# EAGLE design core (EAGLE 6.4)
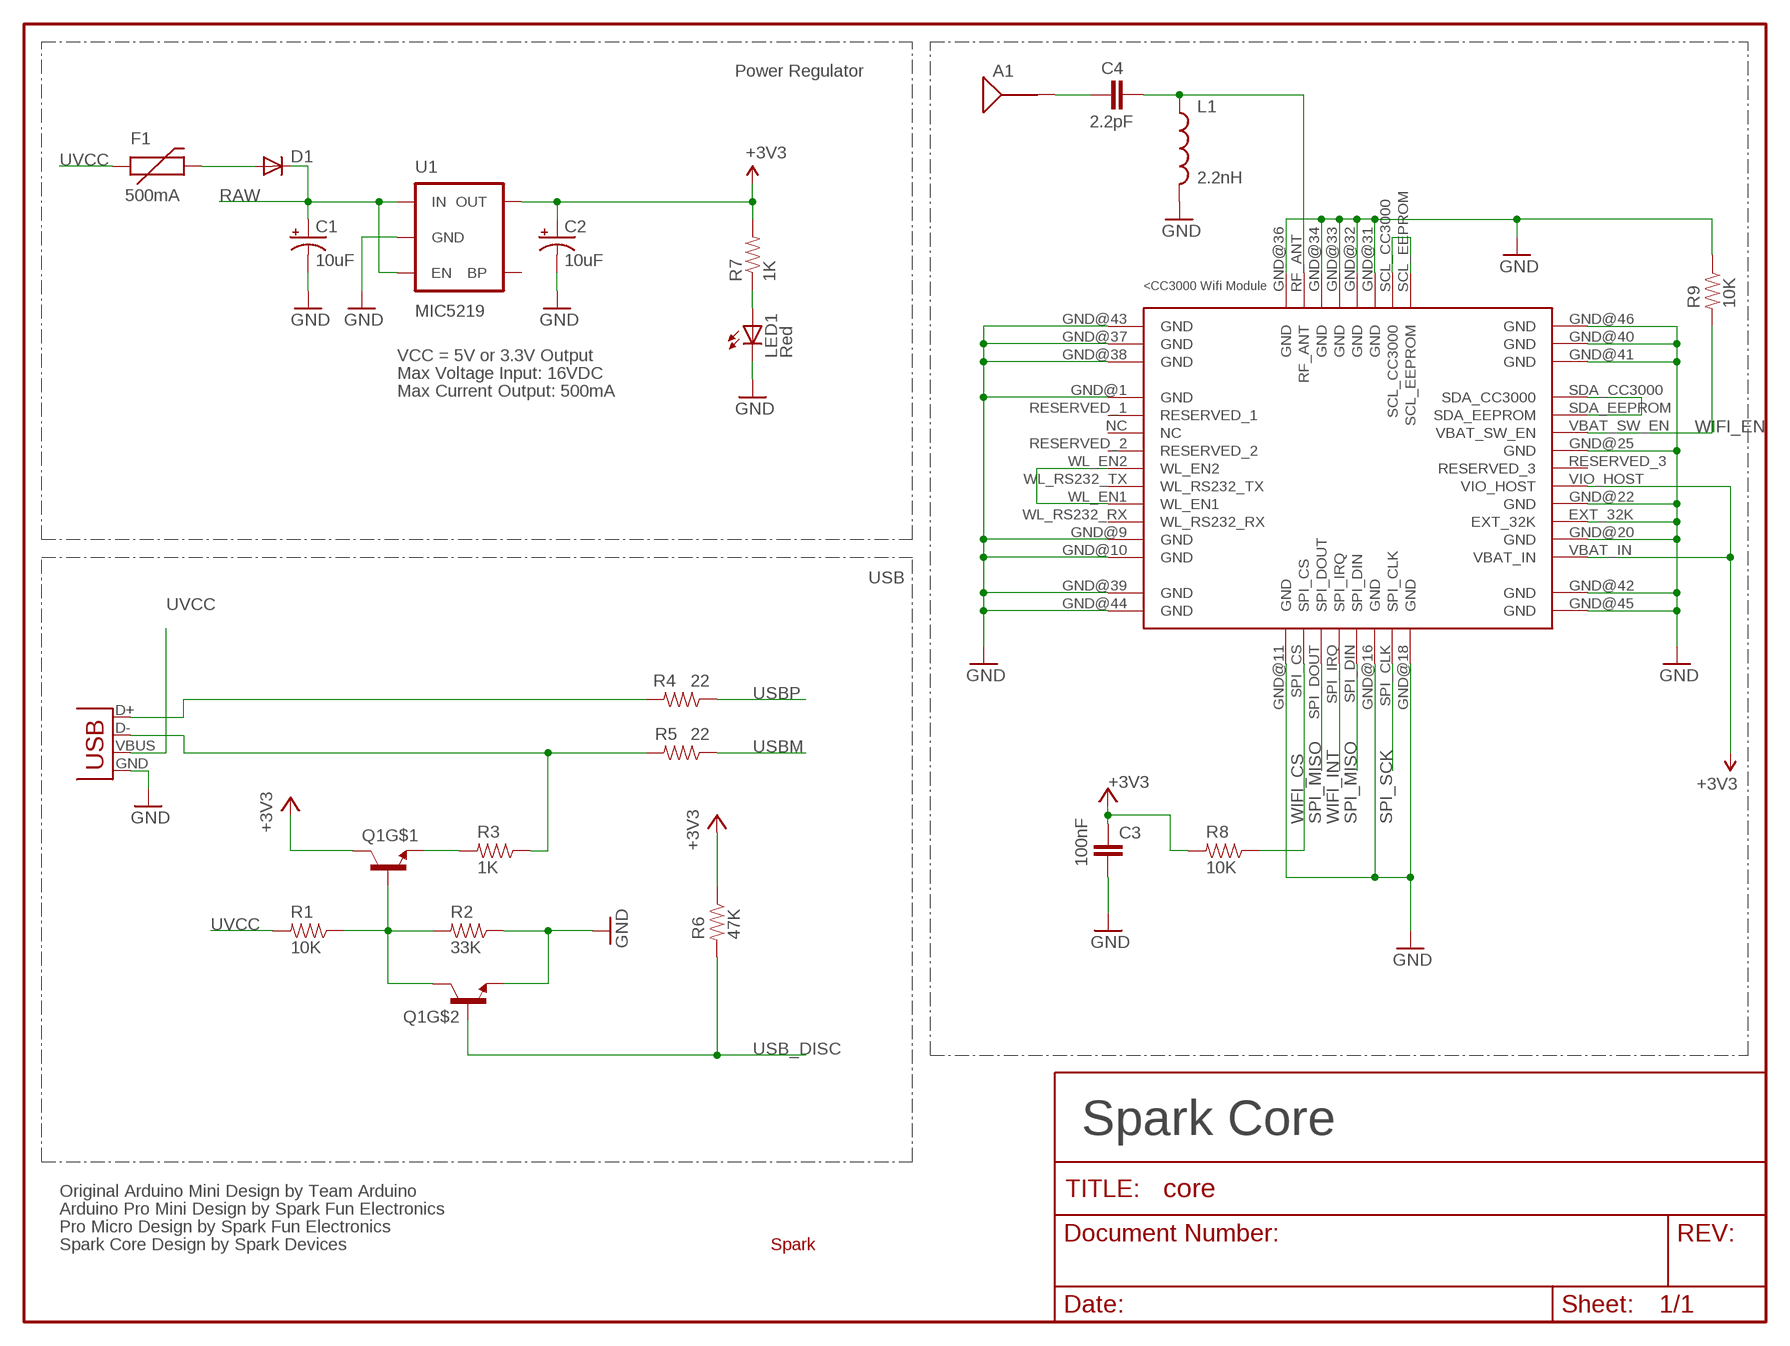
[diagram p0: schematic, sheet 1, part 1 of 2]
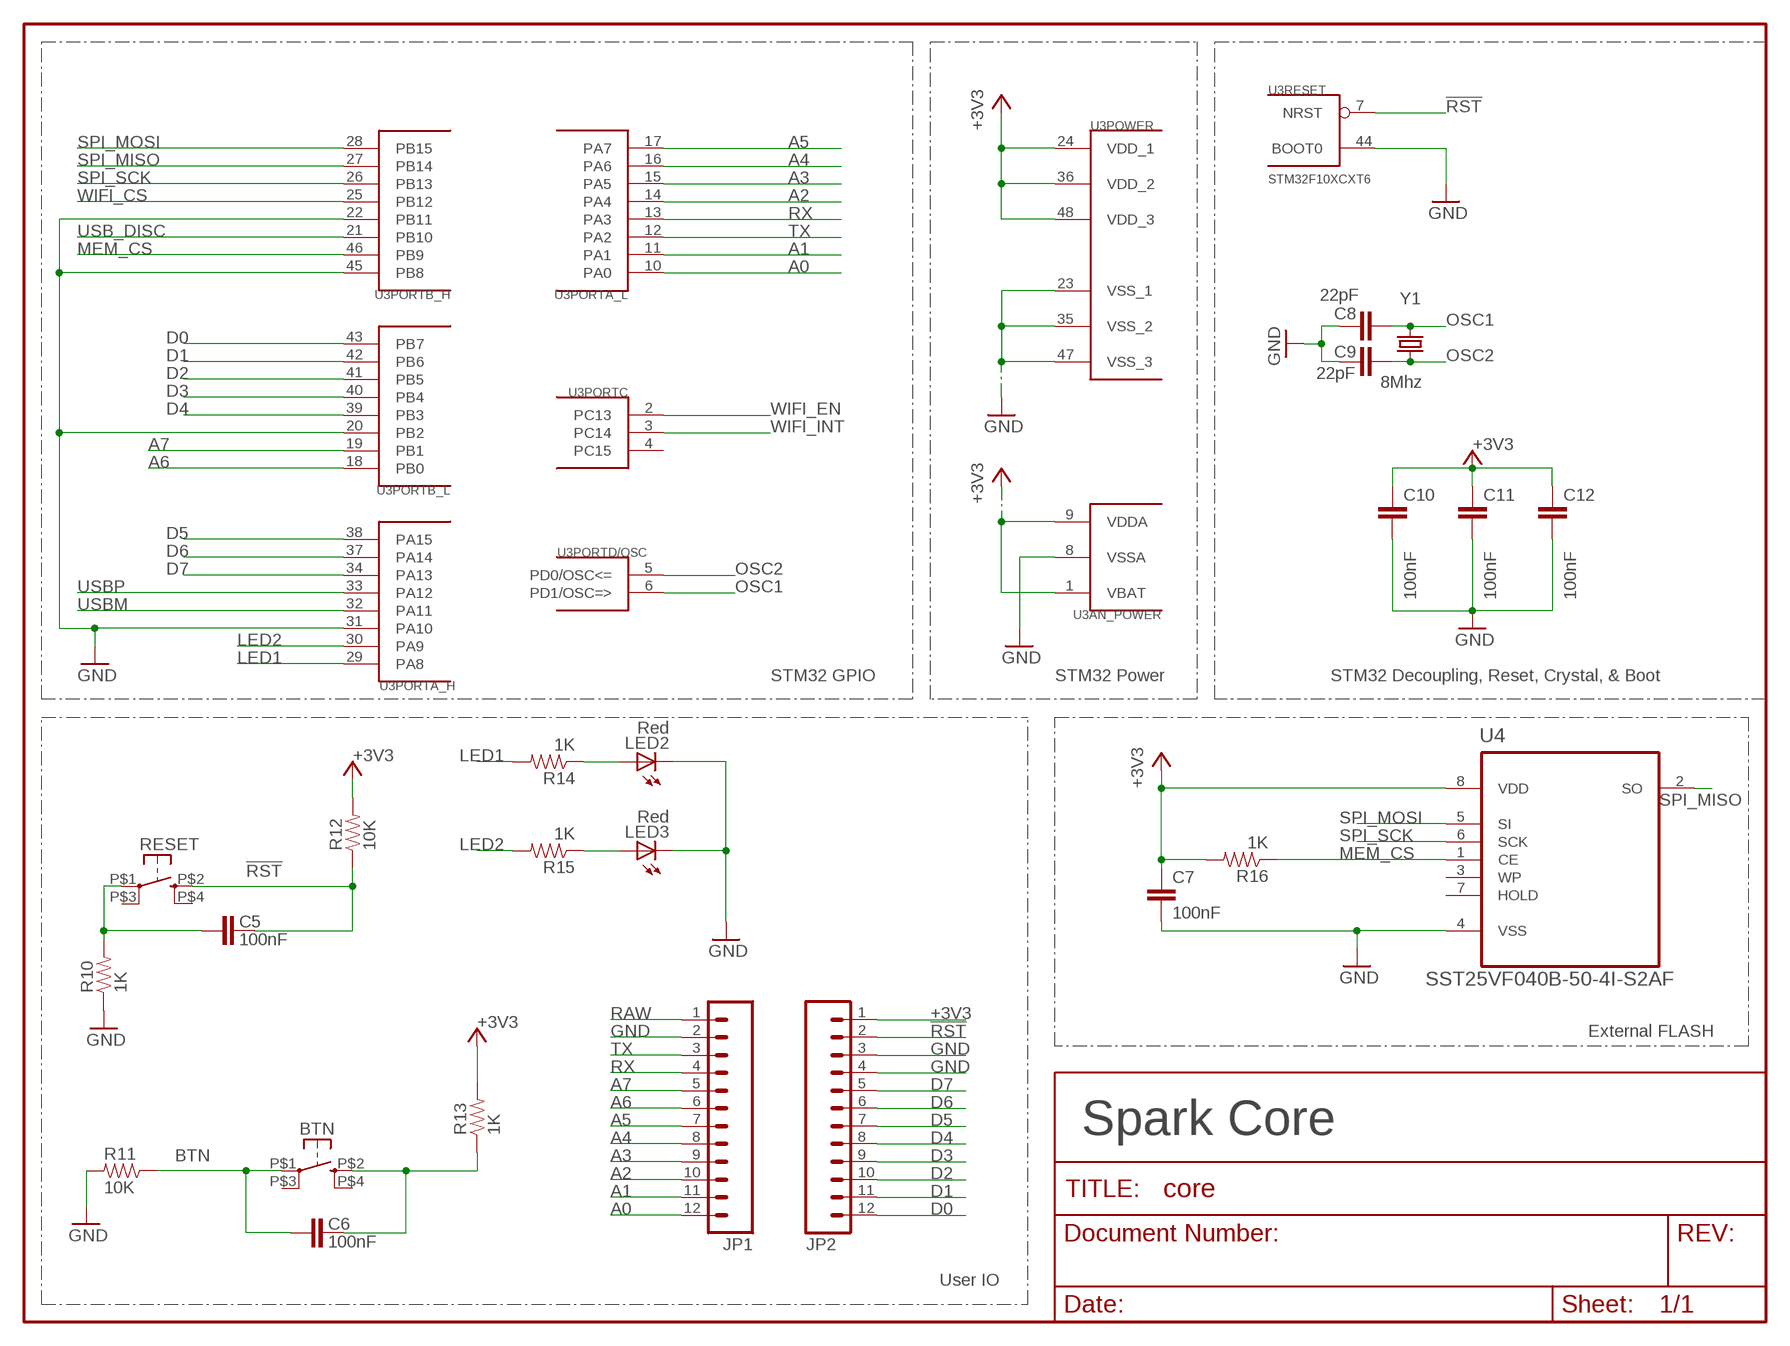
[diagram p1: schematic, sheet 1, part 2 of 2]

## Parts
A1  ANTENNA2SMD5  [ANTENNA-CHIP5]
BTN  KMR211GLFS  BUTTON-KMR241GLFS  [PUSHBUTTON-KMR241GLFS]
C1  10uF  CAP_POL1206  [EIA3216]
C2  10uF  CAP_POL1206  [EIA3216]
C3  100nF  CAP0402-CAP  [0402-CAP]
C4  2.2pF  CAP0402-CAP  [0402-CAP]
C5  100nF  CAP0402-CAP  [0402-CAP]
C6  100nF  CAP0402-CAP  [0402-CAP]
C7  100nF  CAP0402-CAP  [0402-CAP]
C8  22pF  CAP0402-CAP  [0402-CAP]
C9  22pF  CAP0402-CAP  [0402-CAP]
C10  100nF  CAP0402-CAP  [0402-CAP]
C11  100nF  CAP0402-CAP  [0402-CAP]
C12  100nF  CAP0402-CAP  [0402-CAP]
D1  DIODESOD  [SOD-323]
F1  500mA  PTCSMD  [PTC-1206]
JP1  M12PTH  [1X12]
JP2  M12PTH  [1X12]
L1  2.2nH  INDUCTOR0402  [C0402]
LED1  Red  LED0603  [LED-0603]
LED2  Red  LED0603  [LED-0603]
LED3  Red  LED0603  [LED-0603]
Q1  MMDT3904  [SOT363]
R1  10K  RESISTOR0402-RES  [0402-RES]
R2  33K  RESISTOR0402-RES  [0402-RES]
R3  1K  RESISTOR0402-RES  [0402-RES]
R4  22  RESISTOR0402-RES  [0402-RES]
R5  22  RESISTOR0402-RES  [0402-RES]
R6  47K  RESISTOR0402-RES  [0402-RES]
R7  1K  RESISTOR0402-RES  [0402-RES]
R8  10K  RESISTOR0402-RES  [0402-RES]
R9  10K  RESISTOR0402-RES  [0402-RES]
R10  1K  RESISTOR0402-RES  [0402-RES]
R11  10K  RESISTOR0402-RES  [0402-RES]
R12  10K  RESISTOR0402-RES  [0402-RES]
R13  1K  RESISTOR0402-RES  [0402-RES]
R14  1K  RESISTOR0402-RES  [0402-RES]
R15  1K  RESISTOR0402-RES  [0402-RES]
R16  1K  RESISTOR0402-RES  [0402-RES]
RESET  KMR211GLFS  BUTTON-KMR241GLFS  [PUSHBUTTON-KMR241GLFS]
U1  MIC5219  V_REG_LDOSMD  [SOT23-5]
U2  CC3000  [CC3000]
U3  STM32F10XCXT6  [TQFP48]
U4  SST25VF040B-50-4I-S2AF  [SOIC127P790X216-8N]
U$1  SPARK_LOGO2  [SPARK_LOGO2]
X1  USB-MICROB  [USB-MICROB]
Y1  8Mhz  CRYSTAL5X3  [CRYSTAL-SMD-5X3]

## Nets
!RST: C5.2 JP2.2 R12.1 RESET.P$2 U3.7(RESET:NRST)
+3V3: C2.A(+) C3.1 C7.1 C10.1 C11.1 C12.1 JP2.1 Q1.3(C) R6.1 R7.2 R8.2 R12.2 R13.2 R16.2 U1.5(OUT) U2.VBAT_IN U2.VIO_HOST U3.1(AN_POWER:VBAT) U3.9(AN_POWER:VDDA) U3.24(POWER:VDD_1) U3.36(POWER:VDD_2) U3.48(POWER:VDD_3) U4.8(VDD)
A0: JP1.12 U3.10(PORTA_L:PA0)
A1: JP1.11 U3.11(PORTA_L:PA1)
A2: JP1.10 U3.14(PORTA_L:PA4)
A3: JP1.9 U3.15(PORTA_L:PA5)
A4: JP1.8 U3.16(PORTA_L:PA6)
A5: JP1.7 U3.17(PORTA_L:PA7)
A6: JP1.6 U3.18(PORTB_L:PB0)
A7: JP1.5 U3.19(PORTB_L:PB1)
BTN: BTN.P$1 C6.1 R11.1
D0: JP2.12 U3.43(PORTB_L:PB7)
D1: JP2.11 U3.42(PORTB_L:PB6)
D2: JP2.10 U3.41(PORTB_L:PB5)
D3: JP2.9 U3.40(PORTB_L:PB4)
D4: JP2.8 U3.39(PORTB_L:PB3)
D5: JP2.7 U3.38(PORTA_H:PA15)
D6: JP2.6 U3.37(PORTA_H:PA14)
D7: JP2.5 U3.34(PORTA_H:PA13)
GND [vcc]: C1.C(-) C2.C(-) C3.2 C7.2 C8.2 C9.2 C10.2 C11.2 C12.2 JP1.2 JP2.3 JP2.4 L1.2 LED1.C LED2.C LED3.C Q1.1(E) R2.1 R9.1 R10.1 R11.2 U1.2(GND) U2.EXT_32K U2.GND@1(GND) U2.GND@9(GND) U2.GND@10(GND) U2.GND@11(GND) U2.GND@16(GND) U2.GND@18(GND) U2.GND@20(GND) U2.GND@22(GND) U2.GND@25(GND) U2.GND@31(GND) U2.GND@32(GND) U2.GND@33(GND) U2.GND@34(GND) U2.GND@36(GND) U2.GND@37(GND) U2.GND@38(GND) U2.GND@39(GND) U2.GND@40(GND) U2.GND@41(GND) U2.GND@42(GND) U2.GND@43(GND) U2.GND@44(GND) U2.GND@45(GND) U2.GND@46(GND) U3.8(AN_POWER:VSSA) U3.20(PORTB_L:PB2) U3.22(PORTB_H:PB11) U3.23(POWER:VSS_1) U3.31(PORTA_H:PA10) U3.35(POWER:VSS_2) U3.44(RESET:BOOT0) U3.45(PORTB_H:PB8) U3.47(POWER:VSS_3) U4.4(VSS) X1.GND
LED1: R14.2 U3.29(PORTA_H:PA8)
LED2: R15.2 U3.30(PORTA_H:PA9)
MEM_CS: R16.1 U3.46(PORTB_H:PB9) U4.1(CE)
N$1: C5.1 R10.2 RESET.P$1
N$2: LED2.A R14.1
N$3: D1.2(A) F1.2
N$4: C4.2 L1.1 U2.RF_ANT
N$5: A1.FEED(SIGNAL) C4.1
N$6: R3.1 R5.2 X1.D-
N$7: U2.SCL_CC3000 U2.SCL_EEPROM
N$8: R4.2 X1.D+
N$9: U2.WL_EN1 U2.WL_EN2
N$10: LED3.A R15.1
N$13: Q1.5(B) Q1.6(C) R1.1 R2.2
N$14: BTN.P$2 C6.2 R13.1
N$15: U2.SDA_CC3000 U2.SDA_EEPROM
N$16: Q1.4(E) R3.2
N$38: LED1.A R7.1
OSC1: C8.1 U3.6(PORTD/OSC:PD1/OSC=>) Y1.3
OSC2: C9.1 U3.5(PORTD/OSC:PD0/OSC<=) Y1.1
RAW [vcc]: C1.A(+) D1.1(C) JP1.1 U1.1(IN) U1.3(EN)
RX: JP1.4 U3.13(PORTA_L:PA3)
SPI_MISO: U2.SPI_DIN U2.SPI_DOUT U3.27(PORTB_H:PB14) U4.2(SO)
SPI_MOSI: U3.28(PORTB_H:PB15) U4.5(SI)
SPI_SCK: U2.SPI_CLK U3.26(PORTB_H:PB13) U4.6(SCK)
TX: JP1.3 U3.12(PORTA_L:PA2)
USB_DISC: Q1.2(B) R6.2 U3.21(PORTB_H:PB10)
USBM: R5.1 U3.32(PORTA_H:PA11)
USBP: R4.1 U3.33(PORTA_H:PA12)
UVCC: F1.1 R1.2 X1.VBUS
WIFI_CS: R8.1 U2.SPI_CS U3.25(PORTB_H:PB12)
WIFI_EN: R9.2 U2.VBAT_SW_EN U3.2(PORTC:PC13)
WIFI_INT: U2.SPI_IRQ U3.3(PORTC:PC14)
Unconnected: BTN.P$3 BTN.P$4 RESET.P$3 RESET.P$4 U1.4(BP) U2.NC U2.RESERVED_1 U2.RESERVED_2 U2.RESERVED_3 U2.WL_RS232_RX U2.WL_RS232_TX U3.4(PORTC:PC15) U4.3(WP) U4.7(HOLD)

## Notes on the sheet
- Power Regulator
- VCC = 5V or 3.3V Output
- Max Voltage Input: 16VDC
- Max Current Output: 500mA
- USB
- STM32 GPIO | STM32 Power | STM32 Decoupling, Reset, Crystal, & Boot
- External FLASH
- Spark Core | Spark Core
- Original Arduino Mini Design by Team Arduino
- Arduino Pro Mini Design by Spark Fun Electronics
- Pro Micro Design by Spark Fun Electronics
- Spark Core Design by Spark Devices
- User IO

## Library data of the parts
A1 = SparkFun-RF:ANTENNA2: Chip antenna
BTN RESET = okie:BUTTON-KMR241GLFS
C1 C2 = SparkFun:CAP_POL: Capacitor Polarized
C3-C12 = SparkFun-Capacitors:CAP: Capacitor
D1 = SparkFun:DIODE: Diode
F1 = SparkFun:PTC: Resettable Fuse PTC
JP1 JP2 = SparkFun:M12: Header 12 Standard 12-pin 0.1" header. Use with straight break away headers (SKU : PRT-00116), right angle break away headers (PRT-00553), swiss pins (PRT-00743), machine pins (PRT-00117), and female headers (PRT-00115).
L1 = SparkFun-Passives:INDUCTOR: Inductors
LED1-LED3 = SparkFun:LED: LEDs
Q1 = SparkFun-DiscreteSemi:MMDT3904: Dual NPN transistor
R1-R9 R14-R16 = SparkFun:RESISTOR: Resistor
R10-R13 = SparkFun-Passives:RESISTOR: Resistor
U1 = SparkFun:V_REG_LDO: Voltage Regulator LDO Standard 150mA LDO voltage regulator in SOT-23 layout. Micrel part MIC5205. BP (by-pass) pin is used to lower output noise with 470pF cap.
U2 = CC3000:CC3000
U3 = stm32:STM32F10XCXT6: ST STM32F101/103 48pin LQFP
U4 = Silicon_Storage_Tech_By_element14_Batch_1:SST25VF040B-50-4I-S2AF: 4 Mbit SPI Serial Flash; MPN: SST25VF040B-50-4I-S2AF; OC_FARNELL: 1368690; OC_NEWARK: -; PACKAGE: SOIC-8; SUPPLIER: SILICON STORAGE TECHNOLOGY
U$1 = Spark:SPARK_LOGO2
X1 = SparkFun:USB: USB Connectors USB-B-PTH is fully proven SKU : PRT-00139 USB-miniB is fully proven SKU : PRT-00587 USB-A-PCB is untested. USB-A-H is throughly reviewed, but untested. Spark Fun Electronics SKU : PRT-00437 USB-B-SMT is throughly reviewed, but untested. Needs silkscreen touching up. USB-A-S has not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
Y1 = SparkFun:CRYSTAL: Crystals

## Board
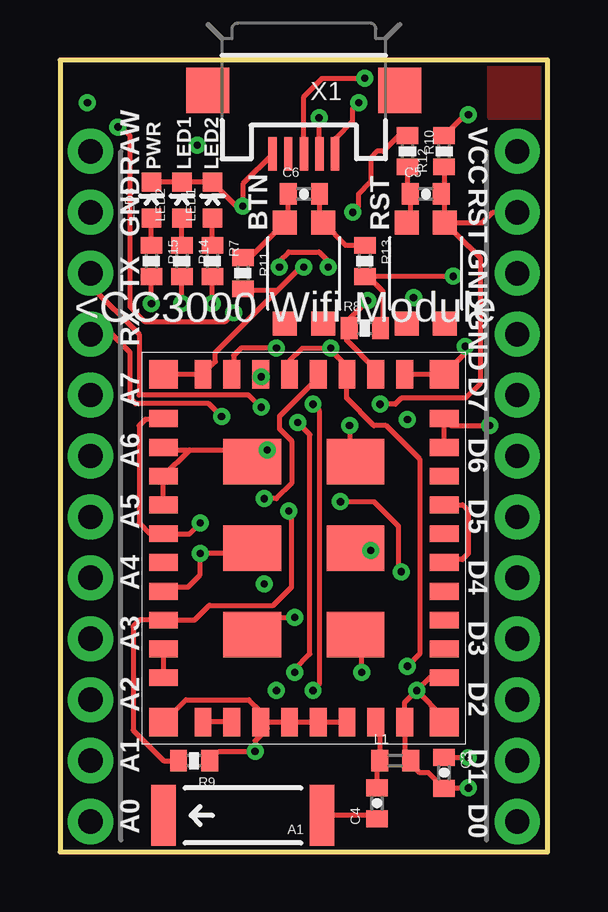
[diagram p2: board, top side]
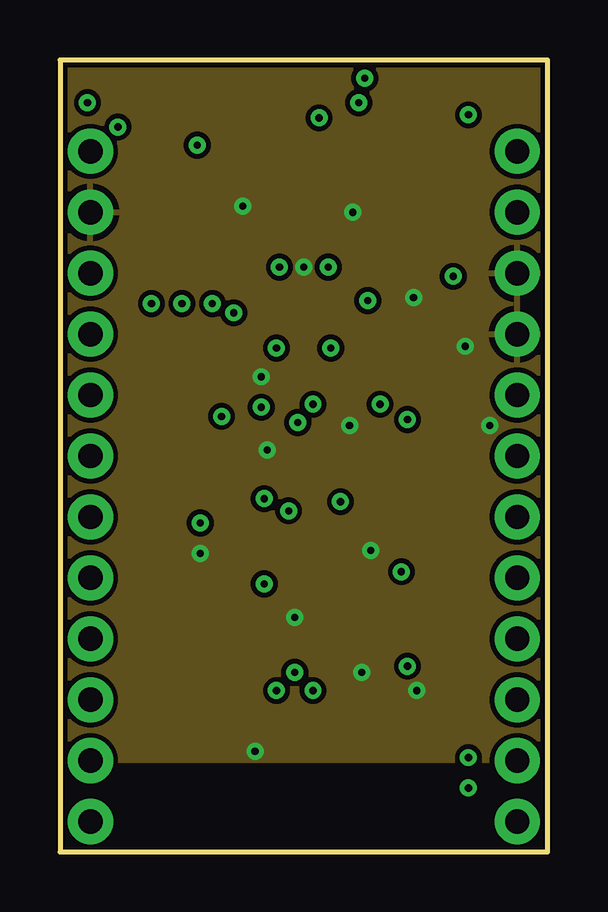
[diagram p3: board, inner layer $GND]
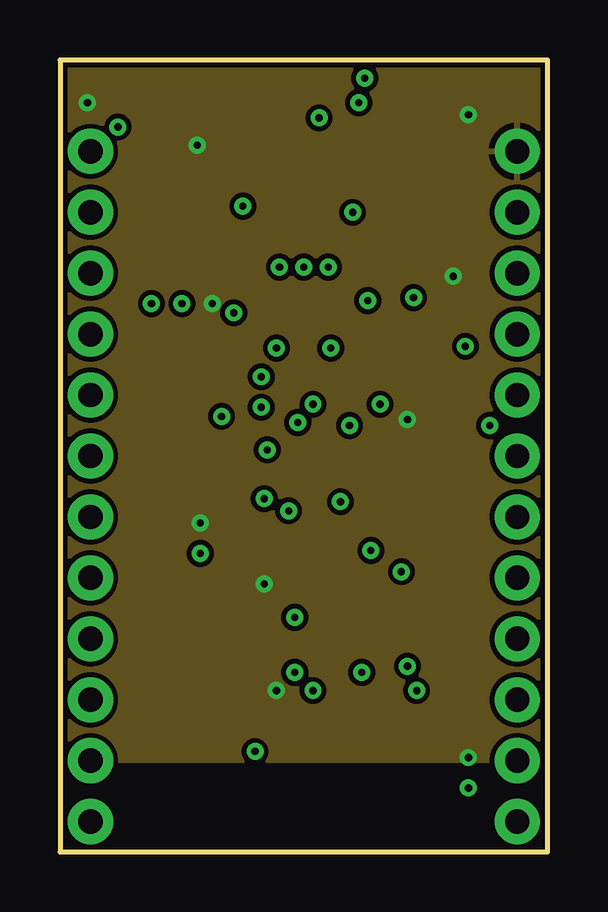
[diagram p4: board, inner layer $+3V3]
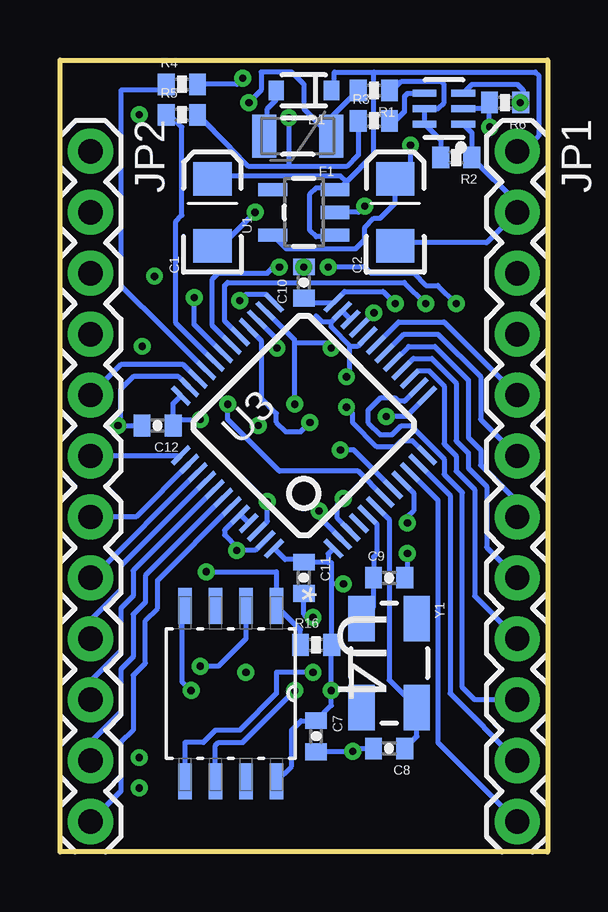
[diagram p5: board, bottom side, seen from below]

Size 20.32 x 33.02 mm. Coordinates in mm from the lower left corner, seen from the top.
Outline: 0,33.02 0,0 20.32,0 20.32,33.02 0,33.02
Copper layers (1+2*15+16): Top 0.035mm / dielectric 1.5mm / $GND 0.035mm / dielectric 0.15mm / $+3V3 0.035mm / dielectric 0.2mm / Bottom 0.035mm
Design rules "default *": minimum track width 6mil, minimum drill 0.3mm, track to track 6mil, track to pad 6mil, pad to pad 6mil, via to via 6mil, smd to smd 6mil, copper to edge 6mil, drill to drill 6mil, minimum pad ring 12mil, minimum via ring 8mil, stop-mask expansion 4mil, vias tented up to drill 20mil, thermal gap 10mil

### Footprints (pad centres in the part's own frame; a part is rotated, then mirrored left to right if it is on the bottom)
ANTENNA-CHIP5 = smd 1.016 x 2.54: FEED -3.302,0; NC 3.302,0
PUSHBUTTON-KMR241GLFS = smd 1 x 1: P$1 2.1,0.8; P$2 2.1,-0.8; P$3 -2.1,0.8; P$4 -2.1,-0.8
EIA3216 = smd 1.4 x 1.6: A 1.4,0; C -1.4,0
0402-CAP = smd 0.7 x 0.9: 1 -0.65,0; 2 0.65,0
SOD-323 = smd 0.63 x 0.83: 1 -1.15,0; 2 1.15,0
PTC-1206 = smd 1 x 1.8: 1 -1.4,0; 2 1.4,0
1X12 = drill 1.016 pad 1.88: 1 0,0; 2 2.54,0; 3 5.08,0; 4 7.62,0; 5 10.16,0; 6 12.7,0; 7 15.24,0; 8 17.78,0; 9 20.32,0; 10 22.86,0; 11 25.4,0; 12 27.94,0
C0402 = smd 0.7 x 0.9: 1 -0.65,0; 2 0.65,0
LED-0603 = smd 0.8 x 0.8: A 0,-0.75; C 0,0.75
SOT363 = smd 0.3 x 0.99: 1 -0.65,-0.8; 2 0,-0.8; 3 0.65,-0.8; 4 0.65,0.81; 5 0,0.81; 6 -0.65,0.81
0402-RES = smd 0.7 x 0.9: 1 -0.65,0; 2 0.65,0
SOT23-5 = smd 0.55 x 1.2: 1 -0.95,-1.3; 2 0,-1.3; 3 0.95,-1.3; 4 0.95,1.3; 5 -0.95,1.3
CC3000 = smd 1.2 x 0.7: EXT_32K 5.85,-2.97; GND@1 -5.85,5.43; GND@9 -5.85,-4.17; GND@10 -5.85,-5.37; GND@20 5.85,-4.17; GND@22 5.85,-1.77; GND@25 5.85,1.83; NC -5.85,3.03; RESERVED_1 -5.85,4.23; RESERVED_2 -5.85,1.83; RESERVED_3 5.85,0.63; SDA_CC3000 5.85,5.43; SDA_EEPROM 5.85,4.23; VBAT_IN 5.85,-5.37; VBAT_SW_EN 5.85,3.03; VIO_HOST 5.85,-0.57; WL_EN1 -5.85,-1.77; WL_EN2 -5.85,0.63; WL_RS232_RX -5.85,-2.97; WL_RS232_TX -5.85,-0.57 | smd 0.7 x 1.2: GND@11 -4.2,-7.22; GND@16 1.8,-7.22; GND@18 4.2,-7.22; GND@31 1.8,7.28; GND@32 0.6,7.28; GND@33 -0.6,7.28; GND@34 -1.8,7.28; GND@36 -4.2,7.28; RF_ANT -3,7.28; SCL_CC3000 3,7.28; SCL_EEPROM 4.2,7.28; SPI_CLK 3,-7.22; SPI_CS -3,-7.22; SPI_DIN 0.6,-7.22; SPI_DOUT -1.8,-7.22; SPI_IRQ -0.6,-7.22 | smd 2.4 x 1.9: GND@37 -2.15,3.63; GND@38 -2.15,0.03; GND@39 -2.15,-3.57; GND@40 2.15,3.63; GND@41 2.15,0.03; GND@42 2.15,-3.57 | smd 1.2 x 1.2: GND@43 -5.85,7.28; GND@44 -5.85,-7.22; GND@45 5.85,-7.22; GND@46 5.85,7.28
TQFP48 = smd 0.2 x 1: 1 -2.75,-4.5; 2 -2.25,-4.5; 3 -1.75,-4.5; 4 -1.25,-4.5; 5 -0.75,-4.5; 6 -0.25,-4.5; 7 0.25,-4.5; 8 0.75,-4.5; 9 1.25,-4.5; 10 1.75,-4.5; 11 2.25,-4.5; 12 2.75,-4.5; 25 2.75,4.5; 26 2.25,4.5; 27 1.75,4.5; 28 1.25,4.5; 29 0.75,4.5; 30 0.25,4.5; 31 -0.25,4.5; 32 -0.75,4.5; 33 -1.25,4.5; 34 -1.75,4.5; 35 -2.25,4.5; 36 -2.75,4.5 | smd 1 x 0.2: 13 4.5,-2.75; 14 4.5,-2.25; 15 4.5,-1.75; 16 4.5,-1.25; 17 4.5,-0.75; 18 4.5,-0.25; 19 4.5,0.25; 20 4.5,0.75; 21 4.5,1.25; 22 4.5,1.75; 23 4.5,2.25; 24 4.5,2.75; 37 -4.5,2.75; 38 -4.5,2.25; 39 -4.5,1.75; 40 -4.5,1.25; 41 -4.5,0.75; 42 -4.5,0.25; 43 -4.5,-0.25; 44 -4.5,-0.75; 45 -4.5,-1.25; 46 -4.5,-1.75; 47 -4.5,-2.25; 48 -4.5,-2.75
SOIC127P790X216-8N = smd 1.499 x 0.559: 1 -3.658,1.905; 2 -3.658,0.635; 3 -3.658,-0.635; 4 -3.658,-1.905; 5 3.658,-1.905; 6 3.658,-0.635; 7 3.658,0.635; 8 3.658,1.905
USB-MICROB = smd 0.35 x 1.4: D+ 0,2.65; D- -0.65,2.65; GND 1.3,2.65; ID 0.65,2.65; VBUS -1.3,2.65 | smd 1.8 x 1.9: MT1 -4,0; MT2 4,0
CRYSTAL-SMD-5X3 = smd 1.9 x 1.1: 1 -1.85,-1.15; 2 1.85,-1.15; 3 1.85,1.15; 4 -1.85,1.15

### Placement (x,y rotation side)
A1  7.62,1.52 180 top
BTN  10.16,24.13 90 top
C1  13.97,26.67 90 bottom
C2  6.35,26.67 90 bottom
C3  16,3.3 270 top
C4  13.21,2.03 90 top
C5  15.24,27.43 0 top
C6  10.16,27.43 0 top
C7  9.65,4.83 270 bottom
C8  6.6,4.32 180 bottom
C9  6.6,11.43 0 bottom
C10  10.16,23.75 90 bottom
C11  10.16,11.43 270 bottom
C12  16.26,17.78 180 bottom
D1  10.16,31.75 180 bottom
F1  10.41,29.84 180 bottom
JP1  1.27,29.21 270 bottom
JP2  19.05,29.21 270 bottom
L1  13.97,3.81 0 top
LED1  6.35,27.18 0 top
LED2  5.08,27.18 0 top
LED3  3.81,27.18 0 top
Q1  4.32,30.99 90 bottom
R1  7.24,31.75 180 bottom
R2  3.81,28.96 180 bottom
R3  7.24,30.48 0 bottom
R4  15.24,32 0 bottom
R5  15.24,30.73 0 bottom
R6  1.78,31.24 180 bottom
R7  6.35,24.64 270 top
R8  12.7,21.84 0 top
R9  5.59,3.81 180 top
R10  14.48,29.21 270 top
R11  7.62,24.13 270 top
R12  16,29.21 90 top
R13  12.7,24.64 270 top
R14  5.08,24.64 270 top
R15  3.81,24.64 270 top
R16  9.65,8.64 0 bottom
RESET  15.24,24.13 90 top
U1  10.16,26.67 90 bottom
U2  10.16,12.7 180 top
U3  10.16,17.78 45 bottom
U4  13.21,6.6 270 bottom
U$1  17.78,30.48 0 top
X1  10.16,31.75 180 top
Y1  6.6,7.87 270 bottom

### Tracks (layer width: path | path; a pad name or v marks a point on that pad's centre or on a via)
!RST  (via drill 0.3)
  Top 0.203: JP2.2 18.03,26.67 17.59,26.23 RESET.P$2 | R12.1 16,27.43 | 16,27.43 C5.2 | 16,27.43 16,26.27 RESET.P$2 | RESET.P$2 17.02,25.25 17.04,25.25 17.53,24.77 17.53,19.56 16.89,18.92 14.22,18.92 13.97,18.67 v13.34,18.67
  Bottom 0.203: v13.34,18.67 13.34,18.03 11.18,15.88 7.9,15.88 U3.7
+3V3  (via drill 0.3)
  Top 0.203: v6.35,22.86 R7.2 6.35,24.13 | v5.84,13.72 5.4,13.27 U2.VIO_HOST 3.75,13.27 3.3,13.72 3.3,17.78 3.56,18.03 4.27,18.03 U2.VBAT_IN | R12.2 16.88,30.73 v17.02,30.73 | R8.2 13.46,21.96 13.46,23.37 12.84,23.99 R13.2 12.46,23.99 12.48,24 v16.38,24 | C3.1 16.02,3.94 v17.02,3.94
  Bottom 0.203: U3.36 15.61,18.7 C12.1 15.35,18.03 v14.48,18.03 | C11.1 10.16,12.19 10.94,12.19 U3.48 | 9.02,11.18 9.02,12.06 9.14,12.06 | 9.02,11.18 9.02,8.62 | 10.16,12.06 C11.1 | 8.97,12.7 U3.1 9.14,12.43 9.14,12.06 | v8.51,11.18 9.02,11.18 | 10.16,11.94 C11.1 | 9.02,8.62 R16.2 | Q1.3 3.15,32 1.27,32 1.02,31.75 1.02,31.24 R6.1 v1.14,31.24 | 9.14,12.06 9.16,12.08 C11.1 | U3.9 5.59,14.98 5.59,14.22 5.84,13.97 v5.84,13.72 | v6.35,22.86 6.86,23.37 8.46,23.37 U3.24 9.97,22.91 C10.1 | v5.71,29.46 5.71,28.7 C2.A 6.35,27.05 6.99,26.42 7.24,26.42 7.62,26.04 7.62,25.53 8,25.15 10.89,25.15 U1.5 | 9.02,8.62 v9.02,6.73 9.02,6.11 C7.1 10.27,5.48 10.67,5.08 10.67,3.58 U4.8
  pour $+3V3 (isolate 0.203): 0,33.02 20.32,33.02 20.32,3.81 0,3.81
A0
  Bottom 0.203: JP1.12 4.57,4.57 4.57,14.67 U3.10
A1
  Bottom 0.203: JP1.11 4.06,6.6 4.06,14.87 U3.11
A2
  Bottom 0.203: JP1.10 3.05,6.35 3.56,6.86 3.56,14.99 4.32,15.75 4.32,16.38 5.71,17.78 6.1,17.78 6.48,17.4 6.99,17.4 7.49,17.91 7.49,18.41 6.99,18.92 6.35,18.92 6.22,18.8 5.96,18.8 U3.14
A3
  Bottom 0.203: JP1.9 3.05,10.67 3.05,15.11 3.81,15.88 3.81,16.51 4.32,17.02 4.32,19.43 4.95,20.07 5.4,20.07 U3.15
A4
  Bottom 0.203: U3.16 5.6,20.57 4.83,20.57 3.81,19.56 3.81,17.14 3.3,16.64 3.3,16 2.54,15.24 2.54,12.7 JP1.8
A5
  Bottom 0.203: JP1.7 1.27,14.61 2.79,16.13 2.79,16.76 3.3,17.27 3.3,19.68 4.7,21.08 5.8,21.08 U3.17
A6
  Bottom 0.203: JP1.6 2.79,18.03 2.79,19.81 4.57,21.59 6,21.59 U3.18
A7
  Bottom 0.203: JP1.5 4.32,22.1 6.22,22.1 6.22,22.07 U3.19
BTN
  Top 0.203: R11.1 7.91,24.78 BTN.P$1 9.51,26.38 C6.1
D0
  Bottom 0.203: U3.43 16.26,11.33 16.26,10.16 16.76,9.65 16.76,7.87 17.27,7.37 17.27,5.08 17.78,4.57 17.78,2.54 JP2.12
D1
  Bottom 0.203: JP2.11 19.05,4.57 17.78,5.84 17.78,7.62 17.27,8.13 17.27,9.91 16.76,10.41 16.76,11.53 U3.42
D2
  Bottom 0.203: JP2.10 19.05,7.11 17.78,8.38 17.78,10.16 17.27,10.67 17.27,11.73 U3.41
D3
  Bottom 0.203: JP2.9 19.05,9.65 17.78,10.92 17.78,11.94 17.77,11.94 U3.40
D4
  Bottom 0.203: U3.39 18.98,11.43 JP2.8
D5
  Bottom 0.203: JP2.7 17.15,13.97 U3.38
D6
  Bottom 0.203: U3.37 15.32,16.51 JP2.6
D7
  Bottom 0.203: JP2.5 17.78,20.32 15.18,20.32 U3.34
GND  (via drill 0.3)
  Top 0.203: 14.48,3.81 L1.2 | v12.19,26.67 12.45,26.92 12.45,27.43 12.95,27.94 12.95,28.96 13.21,29.21 13.46,29.21 14.11,29.86 R10.1 | L1.2 14.36,4.07 U2.GND@36 14.36,6.23 v14.86,6.73 | U2.GND@43 16.01,5.58 v14.86,6.73 | U2.GND@1 15.4,7.27 v14.86,6.73 | v12.57,7.49 12.57,8.81 U2.GND@37 | v12.06,17.78 12.06,16.52 U2.GND@39 | U2.GND@42 8.14,16.27 v8.64,16.76 5.4,16.76 | v8.38,19.81 8.38,19.9 U2.GND@16 | R9.1 6.62,4.19 v8.13,4.19 8.13,4.64 8.64,5.14 U2.GND@31 | U2.GND@31 U2.GND@32 U2.GND@33 U2.GND@34 | U2.GND@46 5.24,6.35 7.87,6.35 8.36,5.86 U2.GND@31 | C3.2 16.14,2.79 | U2.GND@41 7.79,12.45 v5.84,12.45 5.84,11.56 5.33,11.05 4.49,11.05 U2.GND@25 | 5.4,16.76 U2.EXT_32K U2.GND@22 | U2.GND@20 4.42,16.76 5.4,16.76 | U2.GND@45 U2.GND@18 6.48,20.44 6.48,20.83 9.08,23.43 | R11.2 7.73,23.37 7.79,23.43 9.08,23.43 | 9.08,23.43 10.03,24.38 v10.16,24.38 | LED3.C LED2.C LED1.C 7.35,26.92 v7.62,26.92 7.62,27.86 X1.GND | v17.91,17.78 16.3,17.78 U2.GND@10 U2.GND@9 | U2.GND@40 8.72,9.78 v9.78,9.78 | U2.GND@38 12.41,12.57 v12.95,12.57 | v16.89,21.08 16.89,20.8 U2.GND@44 U2.GND@11 | C3.2 16.02,2.67 v17.02,2.67 | C3.2 15.35,3.3 14.99,3.3 14.62,3.67 L1.2
  Bottom 0.203: U3.35 15.37,19.81 17.27,19.81 17.78,19.3 17.78,17.78 | C11.2 10.16,9.91 10.03,9.78 v9.78,9.78 | 9.65,22.35 9.4,22.1 9.02,22.1 | v5.84,12.45 5.84,11.43 C9.2 | 17.78,17.78 C12.2 | 17.78,17.78 v17.91,17.78 | U1.2 7.87,26.67 v7.62,26.92 | C2.C 6.35,25.4 2.54,25.4 JP1.2 1.27,27.07 R2.1 | v12.19,26.67 13.46,25.4 13.97,25.4 C1.C | U3.47 11.8,12.95 11.81,12.95 12.19,12.57 v12.95,12.57 12.95,12.7 13.46,13.21 13.46,13.42 U3.44 U3.45 | U3.8 8.08,16.76 v8.64,16.76 | 9.02,22.1 U3.23 U3.22 | 14.61,21.87 U3.31 14.73,22 v14.73,23.11 | 3.05,28.96 R2.1 | Q1.1 3.16,29.98 R2.1 | U4.4 15.24,10.13 15.24,7.11 v14.86,6.73 | 7.51,4.06 C8.2 8,4.32 v8.13,4.19 | U3.20 7.92,21.08 8.2,21.08 | 9.02,22.1 9.02,21.9 8.2,21.08 | v8.38,19.81 8.26,19.94 8.26,21.08 8.2,21.08 | C10.2 v10.16,24.38 | v8.13,4.19 8.26,4.32 | C7.2 v8.13,4.19
  pour $GND (isolate 0.203): 0,33.02 20.32,33.02 20.32,3.81 0,3.81
LED1  (via drill 0.3)
  Top 0.203: v5.08,22.86 R14.2
  Bottom 0.203: U3.29 13.46,22.14 13.46,23.62 13.34,23.75 5.97,23.75 v5.08,22.86 5.08,23.11
LED2  (via drill 0.3)
  Top 0.203: v3.81,22.86 R15.2 | v9.14,24.38 9.14,24.64 9.53,25.02 10.79,25.02 11.18,24.64 v11.18,24.38
  Bottom 0.203: v3.81,22.86 4.57,23.62 5.08,23.62 5.59,24.13 7.37,24.13 7.62,24.38 v9.14,24.38 | U3.30 13.97,21.94 13.97,23.88 13.72,24.13 11.68,24.13 11.43,24.38 v11.18,24.38
MEM_CS  (via drill 0.3)
  Top 0.203: v14.22,11.68 14.1,11.81 14.1,13.59 13.08,14.61 v11.68,14.61
  Bottom 0.203: v14.22,11.68 11.3,11.68 U4.1 10.3,9.26 R16.1 | U3.46 11.68,13.78 v11.68,14.61
N$1
  Top 0.203: R10.2 14.48,27.54 C5.1 14.59,26.38 RESET.P$1
N$2
  Top 0.203: R14.1 LED2.A
N$3
  Bottom 0.203: 11.43,31.75 D1.2 11.31,31.36 11.68,30.99 11.68,29.98 F1.2
N$4
  Top 0.203: U2.RF_ANT arc-90 13.32,5.26 L1.1 arc90 13.21,3.7 C4.2
N$5
  Top 0.203: C4.1 arc-90 13.1,1.27 12.84,1.52 A1.FEED
N$6  (via drill 0.3)
  Top 0.203: X1.D- 10.79,29.11 v10.79,30.61
  Bottom 0.203: R3.1 7.89,29.48 | 7.89,29.48 7.87,29.46 | 7.89,29.48 7.89,29.07 8.38,28.57 10.79,28.57 | 10.79,28.57 12.45,28.57 13.21,29.34 13.21,29.35 R5.2 | v10.79,30.61 10.79,28.57
N$7
  Top 0.203: U2.SCL_CC3000 U2.SCL_EEPROM
N$8  (via drill 0.3)
  Top 0.203: X1.D+ 10.16,31.5 10.92,32.26 v12.7,32.26
  Bottom 0.203: v12.7,32.26 12.95,32 R4.2
N$9
  Top 0.203: U2.WL_EN1 16.77,14.47 17.02,14.22 17.02,12.45 16.76,12.19 16.13,12.19 U2.WL_EN2
N$10
  Top 0.203: R15.1 LED3.A
N$11
  pour Top: 17.91,33.02 20.32,33.02 20.32,30.61 17.91,30.61
N$13
  Bottom 0.203: R1.1 6.48,31.75 6.1,32.13 4.45,32.13 4.32,32 4.32,31.24 4.57,30.99 Q1.5 Q1.6 4.46,29.67 R2.2
N$14
  Top 0.203: R13.1 11.9,25.29 BTN.P$2 10.81,26.38 C6.2
N$15
  Top 0.203: U2.SDA_EEPROM U2.SDA_CC3000
N$16
  Bottom 0.203: Q1.4 5.14,31.62 5.84,31.62 5.97,31.5 5.97,30.86 6.35,30.48 R3.2
N$38
  Top 0.203: R7.1 LED1.A
OSC1
  Bottom 0.203: 5.97,4.32 C8.1 5.45,4.82 Y1.3 6.6,7.17 6.6,13.87 U3.6
OSC2
  Bottom 0.203: C9.1 | 7.11,11.57 C9.1 | U3.5 7.11,13.67 7.11,12.45 7.25,12.3 C9.1 | Y1.1 7.25,10.22 C9.1
RAW
  Bottom 0.203: 8.89,31.75 8.89,31.5 | 7.24,32.51 8.89,32.51 8.89,31.75 | 7.24,32.51 0.51,32.51 0.38,32.38 0.38,29.84 1.02,29.21 JP1.1 | 8.89,31.75 D1.1 | C1.A 13.97,28.19 8.64,28.19 8.38,27.94 | U1.1 8.93,25.65 9.65,25.65 9.91,25.91 9.91,27.43 9.65,27.69 8.93,27.69 U1.3 8.7,27.62 8.38,27.94 | 8.38,27.94 7.24,29.08 7.24,32.51
RX  (via drill 0.3)
  Top 0.203: JP1.4 2.16,21.59 2.92,20.83 2.92,18.92 3.15,18.69 6.2,18.69 v6.73,18.16
  Bottom 0.203: v6.73,18.16 5.89,18.16 U3.13
SPI_MISO  (via drill 0.3)
  Top 0.203: v14.48,7.75 14.99,8.26 14.99,16.38 13.59,17.78 13.08,17.78 11.94,18.92 11.94,19.9 U2.SPI_DOUT 11.96,20.25 11.28,20.93 v11.28,21.01 10.08,21.01 9.56,20.48 U2.SPI_DIN
  Bottom 0.203: U4.2 12.57,8.89 13.72,7.75 v14.48,7.75 | U3.27 11.28,21.37 v11.28,21.01
SPI_MOSI  (via drill 0.3)
  Top 0.203: v9.78,7.49 9.78,7.62 10.41,8.26 10.41,17.4 v9.91,17.91 10.03,17.78
  Bottom 0.203: U4.5 15.11,4.57 14.35,4.57 13.84,5.08 12.83,5.08 11.3,6.6 11.3,7.49 v9.78,7.49 | v9.91,17.91 10.29,17.53 10.92,17.53 11.3,17.91 11.3,18.29 11.94,18.92 11.94,21.33 U3.28
SPI_SCK  (via drill 0.3)
  Top 0.203: 7.16,20.37 U2.SPI_CLK 7.24,20 7.24,20.7 7.54,21.01 v9.02,21.01 | v10.54,18.67 10.79,18.41 10.79,6.99 v10.54,6.73
  Bottom 0.203: v10.54,18.67 10.54,21.21 | 10.54,21.21 10.54,21.34 U3.26 | v10.54,6.73 12.7,4.57 13.72,4.57 13.84,4.45 U4.6 | v9.02,21.01 9.22,21.21 10.54,21.21
TX  (via drill 0.3)
  Top 0.203: JP1.3 1.27,23.62 3.3,21.59 3.3,19.05 7.87,19.05 v8.38,18.54
  Bottom 0.203: v8.38,18.54 8.13,18.29 8.13,17.91 7.11,16.89 6.35,16.89 6.1,17.14 5.64,17.14 U3.12
USB_DISC  (via drill 0.3)
  Top 0.203: v7.24,22.48 6.86,22.1 3.56,22.1 2.92,22.73 2.92,29.84 2.54,30.23 v2.41,30.23
  Bottom 0.203: Q1.2 2.54,30.99 2.29,31.24 R6.2 2.43,30.24 v2.41,30.23 | U3.21 v7.24,22.47 v7.24,22.48
USBM
  Bottom 0.203: U3.32 15.49,22.05 15.49,26.29 15.24,26.54 15.24,30.23 15.75,30.73 R5.1
USBP
  Bottom 0.203: U3.33 15.99,21.84 16,21.84 17.78,23.62 17.78,31.75 16.14,31.75 R4.1
UVCC  (via drill 0.3 pad 0.41)
  Top 0.203: v12.45,31.24 12.19,30.99 12.19,30.48 11.46,29.75 X1.VBUS
  Bottom 0.203: 12.45,30.99 v12.45,31.24 11.94,31.75 11.94,32.51 10.67,32.51 10.16,32 10.16,30.99 F1.1 9.01,30.62 R1.2
WIFI_CS  (via drill 0.3)
  Top 0.203: U2.SPI_CS 13.16,20.11 11.94,21.34 11.94,21.84 R8.1 12.05,22.21 v12.83,22.99
  Bottom 0.203: 11.38,22.91 U3.25 11.73,23.24 12.57,23.24 v12.83,22.99
WIFI_EN  (via drill 0.3)
  Top 0.203: 4.33,9.65 U2.VBAT_SW_EN | R9.2 4.32,3.81 3.05,5.08 3.05,9.4 3.32,9.67 U2.VBAT_SW_EN | U2.VBAT_SW_EN 5.61,9.67 6.22,10.29 8.89,10.29 9.65,11.05 9.65,14.1 v9.53,14.22
  Bottom 0.203: U3.2 9.53,13.96 v9.53,14.22
WIFI_INT  (via drill 0.3)
  Top 0.203: U2.SPI_IRQ 10.76,19.78 9.14,18.16 9.14,17.65 9.65,17.14 9.65,15.37 9.02,14.73 v8.51,14.73
  Bottom 0.203: U3.3 8.76,13.91 8.76,14.48 v8.51,14.73

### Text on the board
tPlace: VCC | RAW | PWR | LED1 | LED2 | RST | GND | BTN | RST | GND | TX | GND | RX | D7 | A7 | D6 | A6 | D5 | A5 | D4 | A4 | D3 | A3 | D2 | A2 | D1 | A1 | D0 | A0

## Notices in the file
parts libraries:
SparkFun-Capacitors: Licensing: CC v3.0 Share-Alike You are welcome to use this library for commercial purposes.
